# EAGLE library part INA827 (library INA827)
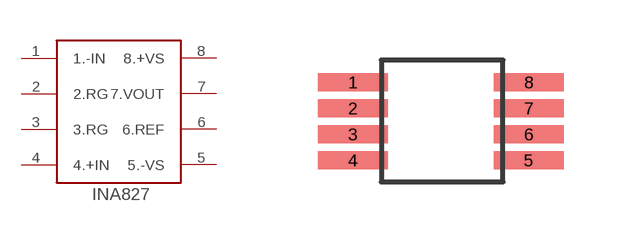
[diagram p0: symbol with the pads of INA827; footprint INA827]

Designator prefix -

## INA827  [INA827]
1  1.-IN
2  2.RG
3  3.RG
4  4.+IN
5  5.-VS
6  6.REF
7  7.VOUT
8  8.+VS

## Footprint INA827 (pad centres in mm)
smd 1.75 x 0.45: 1 -3,3; 2 -3,2.35; 3 -3,1.7; 4 -3,1.05; 5 1.4,1.05; 6 1.4,1.7; 7 1.4,2.35; 8 1.4,3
